FUNCTION_BLOCK FB_LN_IED_LD1_MMXU1 EXTENDS FB_AcsiCommonLogicalNodeClass
VAR_INPUT
	NamPlt: FB_DO_IED_LD1_MMXU1_NamPlt := (sClass:='LPL', bLinkResult:=THIS^.AddDataToContainer(ipData:=NamPlt));
	Beh: FB_DO_IED_LD1_MMXU1_Beh := (sClass:='ENS', bLinkResult:=THIS^.AddDataToContainer(ipData:=Beh));
	Health: FB_DO_IED_LD1_MMXU1_Health := (sClass:='ENS', bLinkResult:=THIS^.AddDataToContainer(ipData:=Health));
	Mod_: FB_DO_IED_LD1_MMXU1_Mod := (sObjectName:='Mod', sClass:='ENC', bLinkResult:=THIS^.AddDataToContainer(ipData:=Mod_));
	TotW: FB_DO_IED_LD1_MMXU1_TotW := (sClass:='MV', bLinkResult:=THIS^.AddDataToContainer(ipData:=TotW));
END_VAR
VAR
END_VAR

END_FUNCTION_BLOCK
